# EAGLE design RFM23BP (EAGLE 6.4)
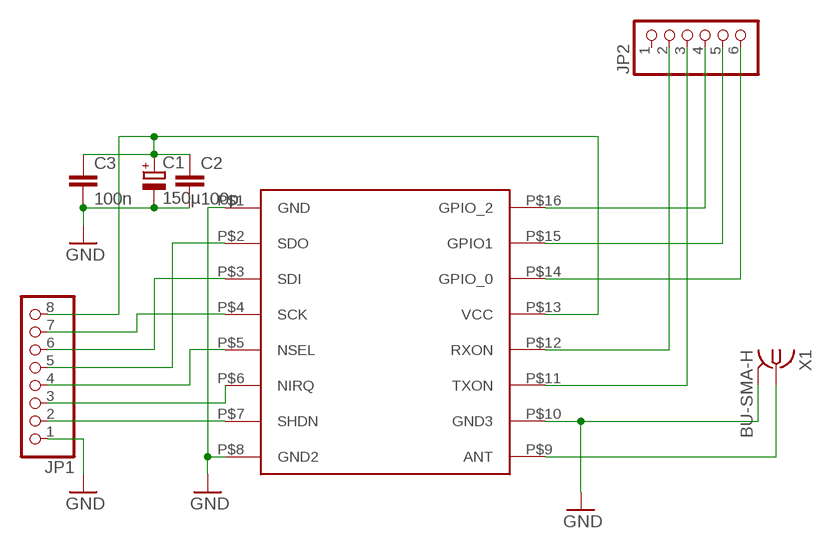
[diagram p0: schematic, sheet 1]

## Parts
C1  150µ  CPOL-EUSMCD  [SMC_D]
C2  100p  C-EUC0805  [C0805]
C3  100n  C-EUC0805  [C0805]
JP1  PINHD-1X8  [1X08]
JP2  PINHD-1X6  [1X06]
U$1  RFM23BP  [RFM23BP]
X1  BU-SMA-H  [BU-SMA-H]

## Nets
GND: C1.- C2.2 C3.2 JP1.1 U$1.P$1(GND) U$1.P$8(GND2) U$1.P$10(GND3) X1.2 X1.3 X1.4 X1.5
N$1: U$1.P$9(ANT) X1.1
N$2: C1.+ C2.1 C3.1 JP1.8 U$1.P$13(VCC)
N$5: JP2.6 U$1.P$14(GPIO_0)
N$6: JP2.5 U$1.P$15(GPIO1)
N$7: JP2.4 U$1.P$16(GPIO_2)
N$8: JP2.2 U$1.P$12(RXON)
N$9: JP2.3 U$1.P$11(TXON)
N$10: JP1.7 U$1.P$4(SCK)
N$11: JP1.6 U$1.P$3(SDI)
N$12: JP1.5 U$1.P$2(SDO)
N$13: JP1.4 U$1.P$5(NSEL)
N$14: JP1.3 U$1.P$6(NIRQ)
N$15: JP1.2 U$1.P$7(SHDN)
Unconnected: JP2.1

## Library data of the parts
C1 = rcl:CPOL-EU: POLARIZED CAPACITOR, European symbol
C2 C3 = rcl:C-EU: CAPACITOR, European symbol
JP1 = pinhead:PINHD-1X8: PIN HEADER
JP2 = pinhead:PINHD-1X6: PIN HEADER
U$1 = RFM23BP_NEW:RFM23BP: RFM23BP module by HopeRF
X1 = con-coax:BU-SMA-H: FEMALE SMA CONNECTOR; OC_FARNELL: unknown; OC_NEWARK: unknown

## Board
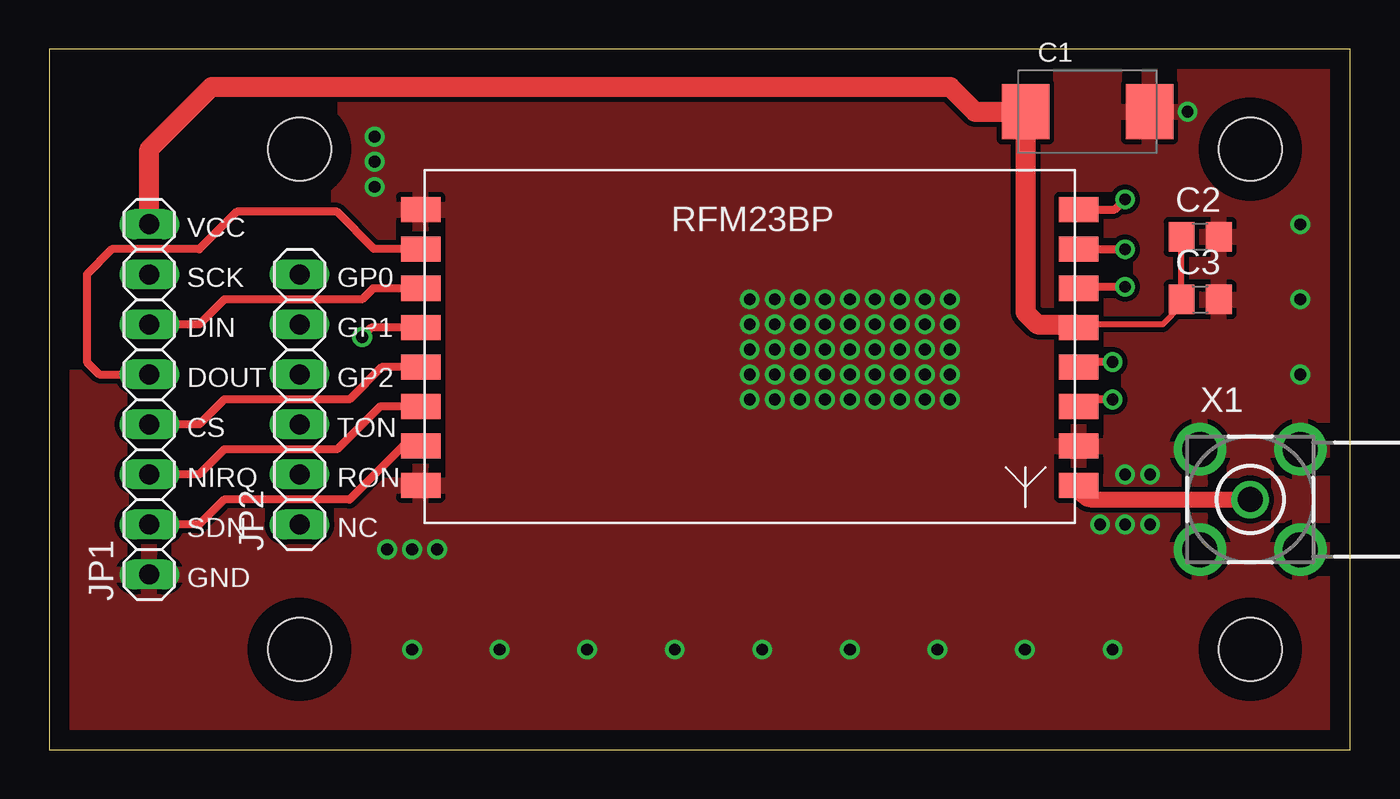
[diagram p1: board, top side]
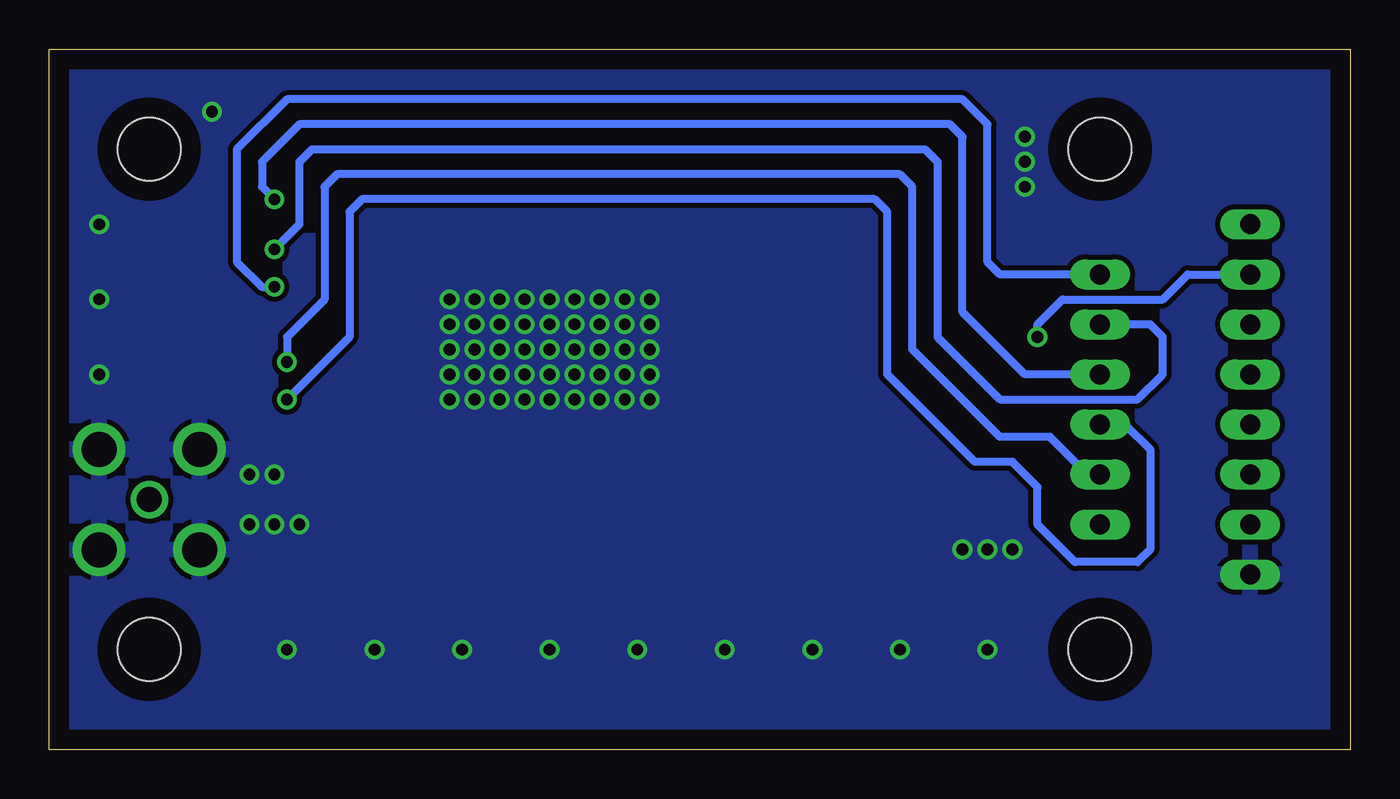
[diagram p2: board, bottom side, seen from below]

Size 66.04 x 35.56 mm. Coordinates in mm from the lower left corner, seen from the top.
Outline: 0,0 66.04,0 66.04,35.56 0,35.56 0,0
Copper layers (1*16): Top 0.035mm / dielectric 1.5mm / Bottom 0.035mm
Design rules "default": minimum track width 10mil, minimum drill 24mil, track to track 8mil, track to pad 8mil, pad to pad 8mil, via to via 8mil, smd to smd 8mil, copper to edge 40mil, drill to drill 8mil, minimum pad ring 10mil, minimum via ring 8mil, stop-mask expansion 4mil, vias tented up to drill 0mil, thermal gap 10mil
Holes 3.2 mm at 12.7,30.48 12.7,5.08 60.96,30.48 60.96,5.08

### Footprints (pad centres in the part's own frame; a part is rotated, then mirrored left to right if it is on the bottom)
SMC_D = smd 2.4 x 2.8: + -3.15,0; - 3.15,0
C0805 = smd 1.3 x 1.5: 1 -0.95,0; 2 0.95,0
1X08 = drill 1.016 long: 1 -8.89,0; 2 -6.35,0; 3 -3.81,0; 4 -1.27,0; 5 1.27,0; 6 3.81,0; 7 6.35,0; 8 8.89,0
1X06 = drill 1.016 long: 1 -6.35,0; 2 -3.81,0; 3 -1.27,0; 4 1.27,0; 5 3.81,0; 6 6.35,0
RFM23BP = smd 2 x 1.27: P$1 -16.7,7.1; P$2 -16.7,5.1; P$3 -16.7,3.1; P$4 -16.7,1.1; P$5 -16.7,-0.9; P$6 -16.7,-2.9; P$7 -16.7,-4.9; P$8 -16.7,-6.9; P$9 16.7,-6.9; P$10 16.7,-4.9; P$11 16.7,-2.9; P$12 16.7,-0.9; P$13 16.7,1.1; P$14 16.7,3.1; P$15 16.7,5.1; P$16 16.7,7.1
BU-SMA-H = drill 1.27: 1 0,0 | drill 1.778: 2 -2.55,2.55; 3 2.55,2.55; 4 2.55,-2.55; 5 -2.55,-2.55

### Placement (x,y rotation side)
C1  52.7,32.38 0 top
C2  58.42,26.04 0 top
C3  58.42,22.86 0 top
JP1  5.08,17.78 90 top
JP2  12.7,17.78 90 top
U$1  35.56,20.32 0 top
X1  60.96,12.7 0 top

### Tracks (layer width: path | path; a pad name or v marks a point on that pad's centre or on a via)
GND  (via drill 0.6)
  other vias: 63.5,26.67 63.5,22.86 63.5,19.05 54.61,13.97 55.88,13.97 53.34,11.43 54.61,11.43 55.88,11.43 18.41,5.08 22.86,5.08 27.3,5.08 31.75,5.08 36.2,5.08 40.64,5.08 45.09,5.08 49.53,5.08 53.98,5.08 45.72,22.86 45.72,21.59 45.72,20.32 45.72,19.05 44.45,22.86 43.18,22.86 41.91,22.86 40.64,22.86 39.37,22.86 38.1,22.86 36.83,22.86 35.56,22.86 35.56,21.59 35.56,21.59 35.56,20.32 35.56,19.05 35.56,19.05 36.83,19.05 36.83,19.05 38.1,19.05 38.1,19.05 39.37,19.05 39.37,19.05 40.64,19.05 40.64,19.05 41.91,19.05 41.91,19.05 43.18,19.05 43.18,19.05 44.45,19.05 36.83,20.32 36.83,21.59 36.83,21.59 38.1,21.59 38.1,21.59 39.37,21.59 39.37,21.59 40.64,21.59 40.64,21.59 41.91,21.59 41.91,21.59 43.18,21.59 43.18,21.59 44.45,21.59 45.72,20.32 44.45,20.32 44.45,20.32 43.18,20.32 41.91,20.32 40.64,20.32 39.37,20.32 38.1,20.32 35.56,17.78 36.83,17.78 38.1,17.78 39.37,17.78 40.64,17.78 41.91,17.78 43.18,17.78 44.45,17.78 45.72,17.78 16.51,31.11 16.51,29.84 57.78,32.38 16.51,28.57 17.14,10.16 18.41,10.16 19.68,10.16
  pour Top (isolate 0.254): 0,35.56 0,0 66.04,0 66.04,35.56
  pour Bottom (isolate 0.254): 0,38.1 68.58,38.1 68.58,-2.54 -2.54,-2.54 -2.54,38.1
N$1
  Top 0.813: U$1.P$9 arc90 52.98,12.7 X1.1
N$2
  Top 0.305: U$1.P$13 52.43,21.59 56.52,21.59 57.47,22.55 C3.1 C2.1
  Top 1.016: JP1.8 5.08,30.48 8.26,33.66 45.72,33.66 46.99,32.38 C1.+ 49.55,22.2 50.16,21.59 52.09,21.59 U$1.P$13
N$5  (via drill 0.6)
  Top 0.406: v54.61,23.5 52.34,23.5 U$1.P$14
  Bottom 0.406: JP2.6 17.78,24.13 18.41,24.77 18.41,31.75 19.68,33.02 53.98,33.02 56.52,30.48 56.52,24.77 55.24,23.5 v54.61,23.5
N$6  (via drill 0.6)
  Top 0.406: U$1.P$15 54.59,25.42 v54.61,25.4
  Bottom 0.406: v54.61,25.4 53.34,26.67 53.34,29.84 52.7,30.48 21.59,30.48 20.95,29.84 20.95,20.95 17.78,17.78 10.79,17.78 9.53,19.05 9.53,20.95 10.16,21.59 JP2.5
N$7  (via drill 0.6)
  Top 0.406: U$1.P$16 54.09,27.42 v54.61,27.94
  Bottom 0.406: JP2.4 16.51,19.05 19.68,22.23 19.68,31.11 20.32,31.75 53.34,31.75 55.24,29.84 55.24,28.57 v54.61,27.94
N$8  (via drill 0.6)
  Top 0.406: v53.98,19.68 52.52,19.68 U$1.P$12
  Bottom 0.406: JP2.2 13.34,13.97 15.24,15.88 17.78,15.88 22.23,20.32 22.23,28.57 22.86,29.21 51.44,29.21 52.07,28.57 52.07,22.86 53.98,20.95 v53.98,19.68
N$9  (via drill 0.6)
  Top 0.406: v53.98,17.78 52.62,17.78 U$1.P$11
  Bottom 0.406: JP2.3 11.43,16.51 10.16,15.24 10.16,10.16 10.79,9.53 13.97,9.53 15.88,11.43 15.88,13.34 17.14,14.61 19.05,14.61 23.5,19.05 23.5,27.3 24.13,27.94 50.16,27.94 50.8,27.3 50.8,20.95 v53.98,17.78
N$10  (via drill 0.6)
  Top 0.406: U$1.P$4 16.34,21.42 v15.88,20.95
  Bottom 0.406: v15.88,20.95 15.88,21.59 14.61,22.86 9.53,22.86 8.26,24.13 JP1.7
N$11
  Top 0.406: U$1.P$3 16.43,23.42 15.88,22.86 8.89,22.86 7.62,21.59 JP1.6
N$12
  Top 0.406: U$1.P$2 16.49,25.42 14.61,27.3 9.53,27.3 7.62,25.4 3.17,25.4 1.91,24.13 1.91,19.68 2.54,19.05 JP1.5
N$13
  Top 0.406: U$1.P$5 16.88,19.42 15.24,17.78 8.89,17.78 7.62,16.51 JP1.4
N$14
  Top 0.406: U$1.P$6 16.79,17.42 14.61,15.24 8.89,15.24 7.62,13.97 JP1.3
N$15
  Top 0.406: U$1.P$7 17.96,15.42 15.24,12.7 8.89,12.7 7.62,11.43 JP1.2

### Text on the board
tPlace: VCC | SCK | GP0 | DIN | GP1 | DOUT | GP2 | CS | TON | NIRQ | RON | SDN | NC | GND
